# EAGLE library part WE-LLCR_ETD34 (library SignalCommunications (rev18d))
WE-LLCR Resonant Converter Characteristics Transformer for high efficiency power supply Input voltage 360–400 VDC Switching frequency 70–120 kHz Output power 150 W–250 W Testing voltage 4 kVAC Litz wire for low eddy current losses Defined leakage inductance for use without additional resonant inductor Applications Power supplies for PC, netbook, LED lighting and other power supplies High efficient resonant converters Details see: http://katalog.we-online.de/en/pbs/WE-LLCR? Updated by Dan Xu 2014-07-07 2014 (C) Wurth Elektronik
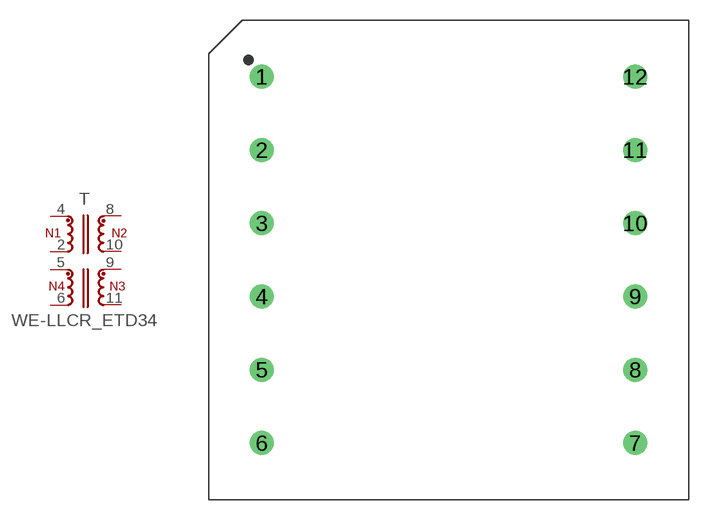
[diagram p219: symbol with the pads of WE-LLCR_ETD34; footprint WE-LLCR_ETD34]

Designator prefix T

## WE-LLCR_ETD34_760895431, WE-LLCR_ETD34_760895441, WE-LLCR_ETD34_760895451  [WE-LLCR_ETD34]
2  8  pas
4  1  pas
5  7  pas
6  6  pas
8  2  pas
9  4  pas
10  3  pas
11  5  pas

## Footprint WE-LLCR_ETD34 (pad centres in mm)
size: ETD34 Height : 26mm max
drill 1.2: 1 -14,13.75; 2 -14,8.25; 3 -14,2.75; 4 -14,-2.75; 5 -14,-8.25; 6 -14,-13.75; 7 14,-13.75; 8 14,-8.25; 9 14,-2.75; 10 14,2.75; 11 14,8.25; 12 14,13.75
